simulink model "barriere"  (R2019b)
settings: Solver=ode45  StartTime=0.0  StopTime=100  RelTol=1e-3  EnableMultiTasking=on
libraries: fl_lib x8, nesl_utility x3, elec_lib x1, simulink x1

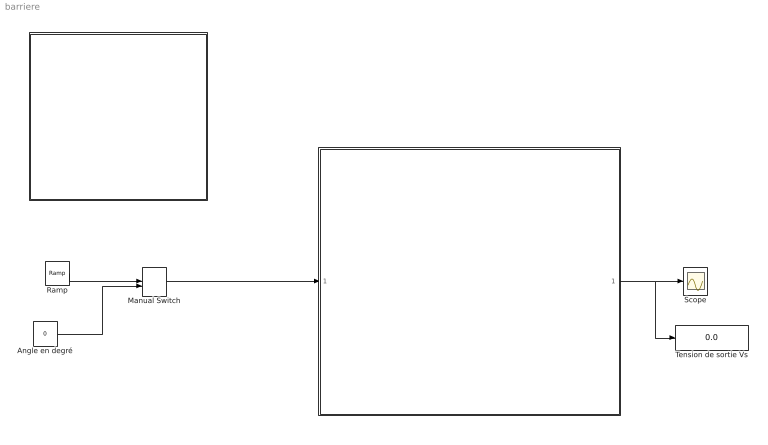
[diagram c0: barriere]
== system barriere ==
  "  " : Subsystem
  "    " : Subsystem
  Angle en degré : Constant  Value=0
  Manual Switch : ManualSwitch
  Ramp : simulink/Sources/Ramp  slope=1  start=0  InitialOutput=0
  Scope : Scope
  Tension de sortie Vs : Display
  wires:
  "  "/1(Out1) -> Scope/1, Tension de sortie Vs/1
  Ramp/1 -> Manual Switch/1
  Manual Switch/1 -> "  "/1(In1)
  Angle en degré/1 -> Manual Switch/2

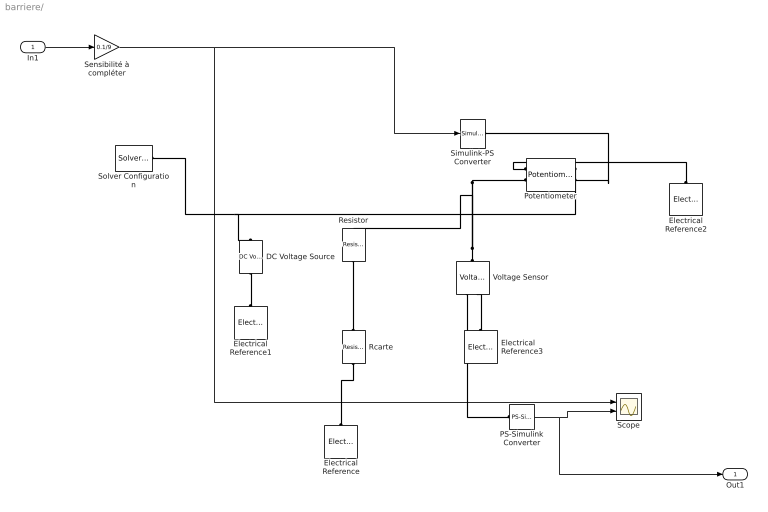
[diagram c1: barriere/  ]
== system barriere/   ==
  In1 : Inport
  DC Voltage Source : fl_lib/Electrical/Electrical Sources/DC Voltage Source  v0=10 V  i_Log=off  v_Log=off  LocalVarNames=|i|v  LocalVarDescs=|i|v  LocalVarLogging=[0 0]
  Electrical Reference{,1..3} (4 alike) : fl_lib/Electrical/Electrical Elements/Electrical Reference  i_Log=off  LocalVarNames=|v1  LocalVarDescs=|v1  LocalVarLogging=[]
  PS-Simulink Converter : nesl_utility/PS-Simulink Converter  PhysicalDomain=network_engine_domain  LeftPortType=input  RightPortType=output  SubClassName=ps_output  Unit=V  AffineConversion=off
  Potentiometer : elec_lib/Passive Devices/Potentiometer  R0=3850 Ohm  Rw=1 Ohm  Rcenter=200 Ohm  xmin=0  xmax=1  Taper=1  Gradient=1  LocalVarLogging=[]
  Rcarte : fl_lib/Electrical/Electrical Elements/Resistor  R=30000 Ohm  i_Log=off  v_Log=off  LocalVarNames=|i|v  LocalVarDescs=|i|v  LocalVarLogging=[0 0]
  Resistor : fl_lib/Electrical/Electrical Elements/Resistor  R=1700 Ohm  i_Log=off  v_Log=off  LocalVarNames=|i|v  LocalVarDescs=|i|v  LocalVarLogging=[0 0]
  Scope : Scope  NumInputPorts=2
  Sensibilité à compléter : Gain  Gain=0.1/9
  Simulink-PS Converter : nesl_utility/Simulink-PS Converter  PhysicalDomain=network_engine_domain  LeftPortType=input  RightPortType=output  SubClassName=ps_input  Unit=1  AffineConversion=off  InputFilterTimeConstant=.001  UdotUserProvided=[]  SimscapeFilterOrder=1  InputFiltering=off
  Solver Configuration : nesl_utility/Solver Configuration  PhysicalDomain=network_engine_domain  LeftPortType=input  RightPortType=generic  SubClassName=solver  UseCustomDae=off  DoDC=on  ResidualTolerance=1e-9  UseLocalSolver=on  LocalSolverChoice=NE_BACKWARD_EULER_ADVANCER  LocalSolverSampleTime=.001  DoFixedCost=on  MaxNonlinIter=3  MaxModeIter=2  LinearAlgebra=Full  Accelerate=off  Profile=off  UseLocalSampling=off  DelaysMemoryBudget=1024
  Voltage Sensor : fl_lib/Electrical/Electrical Sensors/Voltage Sensor  i1_Log=off  v1_Log=off  LocalVarNames=|i1|v1  LocalVarDescs=|i1|v1  LocalVarLogging=[0 0]
  Out1 : Outport
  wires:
  Sensibilité à compléter/1 -> Scope/1, Simulink-PS Converter/1
  PS-Simulink Converter/1 -> Scope/2, Out1/1
  In1/1 -> Sensibilité à compléter/1
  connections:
  Potentiometer/RConn1 -- Solver Configuration/RConn1 -- DC Voltage Source/LConn1
  Voltage Sensor/LConn1 -- Resistor/LConn1 -- Potentiometer/LConn2
  Electrical Reference3/LConn1 -- Voltage Sensor/RConn2
  Voltage Sensor/RConn1 -- PS-Simulink Converter/LConn1
  Rcarte/RConn1 -- Electrical Reference/LConn1
  Resistor/RConn1 -- Rcarte/LConn1
  Electrical Reference1/LConn1 -- DC Voltage Source/RConn1
  Simulink-PS Converter/RConn1 -- Potentiometer/RConn2
  Electrical Reference2/LConn1 -- Potentiometer/LConn1

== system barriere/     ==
